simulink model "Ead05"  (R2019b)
settings: Solver=FixedStepDiscrete  StartTime=0.0  StopTime=20  FixedStep=1  RelTol=1e-3

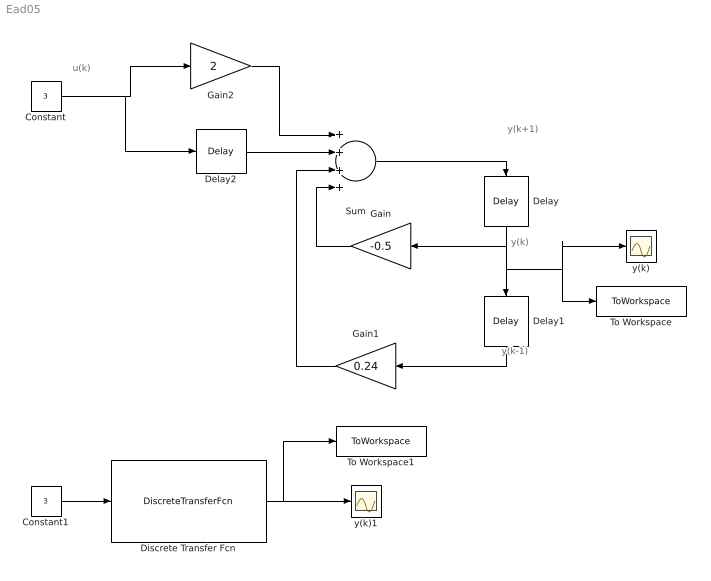
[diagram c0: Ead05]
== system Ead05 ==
  note: y(k+1)
  note: y(k)
  note: y(k-1)
  note: u(k)
  Constant : Constant  Value=3
  Constant1 : Constant  Value=3
  Delay : Delay  DelayLength=1  InitialCondition=2
  Delay1 : Delay  DelayLength=1  InitialCondition=-4.16
  Delay2 : Delay  DelayLength=1  InitialCondition=0
  Discrete Transfer Fcn : DiscreteTransferFcn  Numerator=[2 1]  Denominator=[1 0.5 -0.24]  InitialStates="[3.08  -4.16]"
  Gain : Gain  Gain=-0.5
  Gain1 : Gain  Gain=0.24
  Gain2 : Gain  Gain=2
  Sum : Sum  Inputs=++++
  To Workspace : ToWorkspace  VariableName=y  SaveFormat=Timeseries  SampleTime=-1
  To Workspace1 : ToWorkspace  VariableName=y_DTF1  SaveFormat=Timeseries  SampleTime=-1
  y(k) : Scope
  y(k)1 : Scope
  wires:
  Delay/1 -> Delay1/1, To Workspace/1, y(k)/1, Gain/1
  Sum/1 -> Delay/1
  Delay1/1 -> Gain1/1
  Constant/1 -> Gain2/1, Delay2/1
  Gain2/1 -> Sum/1
  Delay2/1 -> Sum/2
  Gain/1 -> Sum/4
  Gain1/1 -> Sum/3
  Discrete Transfer Fcn/1 -> To Workspace1/1, y(k)1/1
  Constant1/1 -> Discrete Transfer Fcn/1
